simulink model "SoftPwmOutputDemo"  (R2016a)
settings: Solver=FixedStepAuto  StartTime=0.0  StopTime=10.0  RelTol=1e-3
undefined symbols (not defined in the file or in its folder): intmax, Rec, SDTV, strel
libraries: simulink x4, visionstatistics x1, visionconversions x1, visionmorphops x1, embdlinuxlib x1

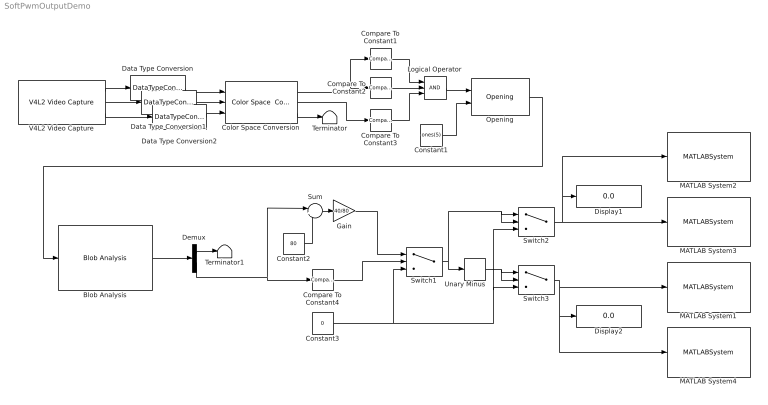
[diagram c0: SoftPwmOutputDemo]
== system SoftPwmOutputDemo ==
  Blob Analysis : visionstatistics/Blob Analysis  Tag=vipblks_row_conv  area=off  centroid=on  bBox=off  majorAxis=off  minorAxis=off  angle=off  eccentricity=off  equivDiameterSq=off  extent=off  perimeter=off  maxBlobs=1  warnIfNumBlobsExceeded=on  isCount=off  useMinArea=off  minArea=0  useMaxArea=off  maxArea=intmax('uint32')  excludeBorderBlob=off  outDT=double  isOutVarDim=off  isFill=on  fillValues=-1  conn=8  isLabel=off  outputMode=Binary point scaling  outputWordLength=32  outputFracLength=16  firstCoeffMode=Binary point scaling  firstCoeffWordLength=16  firstCoeffFracLength=14  secondCoeffMode=Binary point scaling  secondCoeffWordLength=32  secondCoeffFracLength=16  accumMode=Binary point scaling  accumWordLength=32  accumFracLength=0  prodOutputMode=Binary point scaling  prodOutputWordLength=32  prodOutputFracLength=16  roundingMode=Floor  overflowMode=off
  Color Space Conversion : visionconversions/Color Space  Conversion  conversion=Obsolete  conversionActive=R'G'B' to HSV  wp_str=D65  rec=Rec. 601 (SDTV)  sys=1125/60/2:1  imagePorts=Separate color signals
  Compare To Constant1 : simulink/Logic and Bit Operations/Compare To Constant  relop=>=  const=0.5  OutDataTypeStr=boolean
  Compare To Constant2 : simulink/Logic and Bit Operations/Compare To Constant  relop=<=  const=0.7  OutDataTypeStr=boolean
  Compare To Constant3 : simulink/Logic and Bit Operations/Compare To Constant  relop=>=  const=0.8  OutDataTypeStr=boolean
  Compare To Constant4 : simulink/Logic and Bit Operations/Compare To Constant  relop=>=  const=0  OutDataTypeStr=boolean
  Constant1 : Constant  Value=ones(5)  OutDataTypeStr=boolean
  Constant2 : Constant  Value=80  OutDataTypeStr=single
  Constant3 : Constant  Value=0  OutDataTypeStr=single
  Data Type Conversion : DataTypeConversion  OutDataTypeStr=single
  Data Type Conversion1 : DataTypeConversion  OutDataTypeStr=single
  Data Type Conversion2 : DataTypeConversion  OutDataTypeStr=single
  Demux : Demux  Outputs=2
  Display1 : Display
  Display2 : Display
  Gain : Gain  Gain=40/80  OutDataTypeStr=double
  Logical Operator : Logic  Inputs=3  AllPortsSameDT=off  OutDataTypeStr=boolean
  MATLAB System1 : MATLABSystem  System=SoftPwmOutput  Pin=19  InitialValue=0  PwmRange=100
  MATLAB System2 : MATLABSystem  System=SoftPwmOutput  Pin=20  InitialValue=0  PwmRange=100
  MATLAB System3 : MATLABSystem  System=SoftPwmOutput  Pin=21  InitialValue=0  PwmRange=100
  MATLAB System4 : MATLABSystem  System=SoftPwmOutput  Pin=26  InitialValue=0  PwmRange=100
  Opening : visionmorphops/Opening  nhoodsrc=Input port  strel=strel('disk',5)
  Sum : Sum  Inputs=|+-
  Switch1 : Switch  Criteria=u2 > Threshold
  Switch2 : Switch  Criteria=u2 > Threshold  OutDataTypeStr=uint8
  Switch3 : Switch  Criteria=u2 > Threshold  OutDataTypeStr=uint8
  Terminator : Terminator
  Terminator1 : Terminator
  Unary Minus : UnaryMinus
  V4L2 Video Capture : embdlinuxlib/V4L2 Video Capture  m_devName='/dev/video0'  roi=[0, 0, 640, 480]  imSizeSelection=160x120  imSize=[640, 480]  pixelFormat=RGB  pixelOrder=Planar  sampleTime=1/10  simOutput=Colorbars  blockPlatform=Raspberry Pi
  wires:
  V4L2 Video Capture/1 -> Data Type Conversion/1
  V4L2 Video Capture/2 -> Data Type Conversion1/1
  V4L2 Video Capture/3 -> Data Type Conversion2/1
  Color Space Conversion/1 -> Compare To Constant2/1, Compare To Constant1/1
  Compare To Constant1/1 -> Logical Operator/1
  Compare To Constant2/1 -> Logical Operator/2
  Logical Operator/1 -> Opening/1
  Color Space Conversion/2 -> Compare To Constant3/1
  Color Space Conversion/3 -> Terminator/1
  Compare To Constant3/1 -> Logical Operator/3
  Blob Analysis/1 -> Demux/1
  Constant1/1 -> Opening/2
  Sum/1 -> Gain/1
  Constant2/1 -> Sum/2
  Compare To Constant4/1 -> Switch1/2
  Constant3/1 -> Switch1/3, Switch3/3, Switch2/3
  Switch2/1 -> Display1/1, MATLAB System2/1, MATLAB System3/1
  Switch3/1 -> MATLAB System4/1, Display2/1, MATLAB System1/1
  Data Type Conversion/1 -> Color Space Conversion/1
  Data Type Conversion1/1 -> Color Space Conversion/2
  Data Type Conversion2/1 -> Color Space Conversion/3
  Demux/1 -> Terminator1/1
  Demux/2 -> Sum/1, Compare To Constant4/1
  Opening/1 -> Blob Analysis/1
  Unary Minus/1 -> Switch3/2, Switch3/1
  Switch1/1 -> Unary Minus/1, Switch2/2, Switch2/1
  Gain/1 -> Switch1/1
